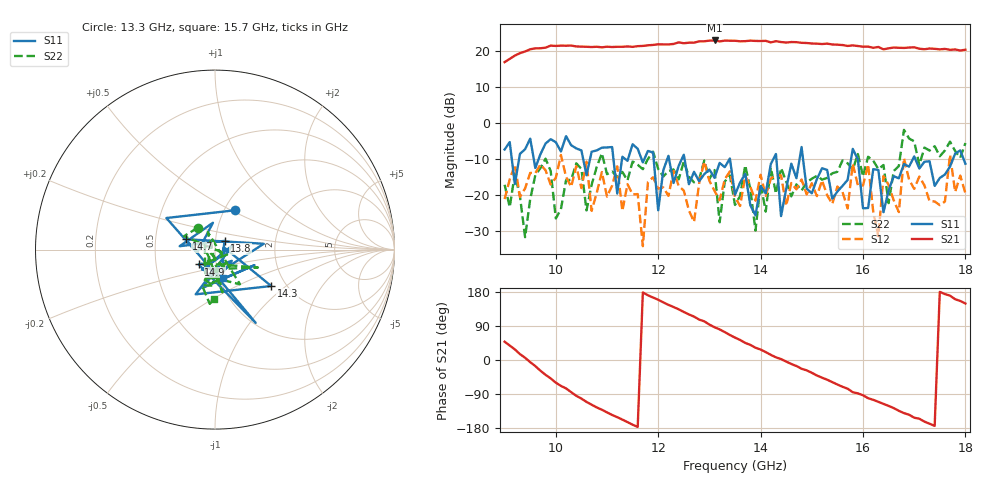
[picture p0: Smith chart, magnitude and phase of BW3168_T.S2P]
!Keysight Technologies,N5247A,US51370447,A.10.64.09
!Date: Saturday, October 09, 2021 21:59:36
!Correction: S11(Full 2 Port with power(1,2))
!S21(Full 2 Port with power(1,2))
!S12(Full 2 Port with power(1,2))
!S22(Full 2 Port with power(1,2))
!S2P File: Measurements: S11, S21, S12, S22:
# Hz S  dB  R 50
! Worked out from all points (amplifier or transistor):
!   91 points, 9 GHz to 18 GHz, reference 50 ohm
!   highest |S21| = 23.0 dB at 13.1 GHz (marker M1)
!   |S21| within 3 dB of that: 9.409 GHz to end of sweep
!   unconditionally stable (mu >= 1): 11.63 GHz to 11.76 GHz; 12.62 GHz to 12.73 GHz; 16.19 GHz to 16.36 GHz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
!   at 10.5 GHz: K = 1.09, MSG = 19.7 dB, |S12| = -18.1 dB
!   at 13.5 GHz: K = 1.03, MSG = 21.7 dB, |S12| = -20.5 dB
!   at 18 GHz: K = 0.80, MSG = 20.0 dB, |S12| = -19.5 dB
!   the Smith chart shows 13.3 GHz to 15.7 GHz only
!   S11 on the Smith chart (normalised r, x): 13.3 GHz: 1.12, +0.52; 13.8 GHz: 1.11, +0.11; 14.3 GHz: 1.68, -0.79; 14.7 GHz: 0.72, +0.09; 14.9 GHz: 0.82, -0.14; 15.7 GHz: 1.03, -0.33
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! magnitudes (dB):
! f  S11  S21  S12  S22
! 9 GHz  -7.3  17.0  -21.1  -17.1
! 9.4 GHz  -7.2  19.9  -18.1  -31.7
! 9.8 GHz  -5.6  21.0  -13.1  -9.9
! 10 GHz  -5.3  21.5  -15.2  -26.5
! 10.5 GHz  -7.6  21.3  -18.1  -12.7
! 11.2 GHz  -19.6  21.2  -12.0  -14.9
! 11.7 GHz  -10.9  21.5  -34.2  -12.8
! 12 GHz  -24.2  21.9  -18.2  -12.7
! 12.2 GHz  -9.1  21.9  -20.2  -13.3
! 13.1 GHz  -15.2  23.0  -18.8  -13.0
! 13.3 GHz  -12.2  22.9  -15.6  -16.2
! 13.5 GHz  -19.9  22.9  -20.5  -22.7
! 13.8 GHz  -22.8  23.0  -17.7  -18.3
! 14.3 GHz  -8.6  22.8  -14.5  -19.5
! 14.4 GHz  -25.8  22.6  -14.5  -12.5
! 14.7 GHz  -15.3  22.5  -18.4  -17.0
! 14.9 GHz  -18.2  22.3  -19.8  -16.5
! 15 GHz  -19.5  22.2  -16.7  -15.4
! 15.7 GHz  -15.8  21.5  -23.7  -11.2
! 16.5 GHz  -18.7  20.8  -17.1  -22.2
! 16.8 GHz  -11.3  20.9  -9.7  -1.9
! 18 GHz  -11.3  20.4  -19.5  -5.5
